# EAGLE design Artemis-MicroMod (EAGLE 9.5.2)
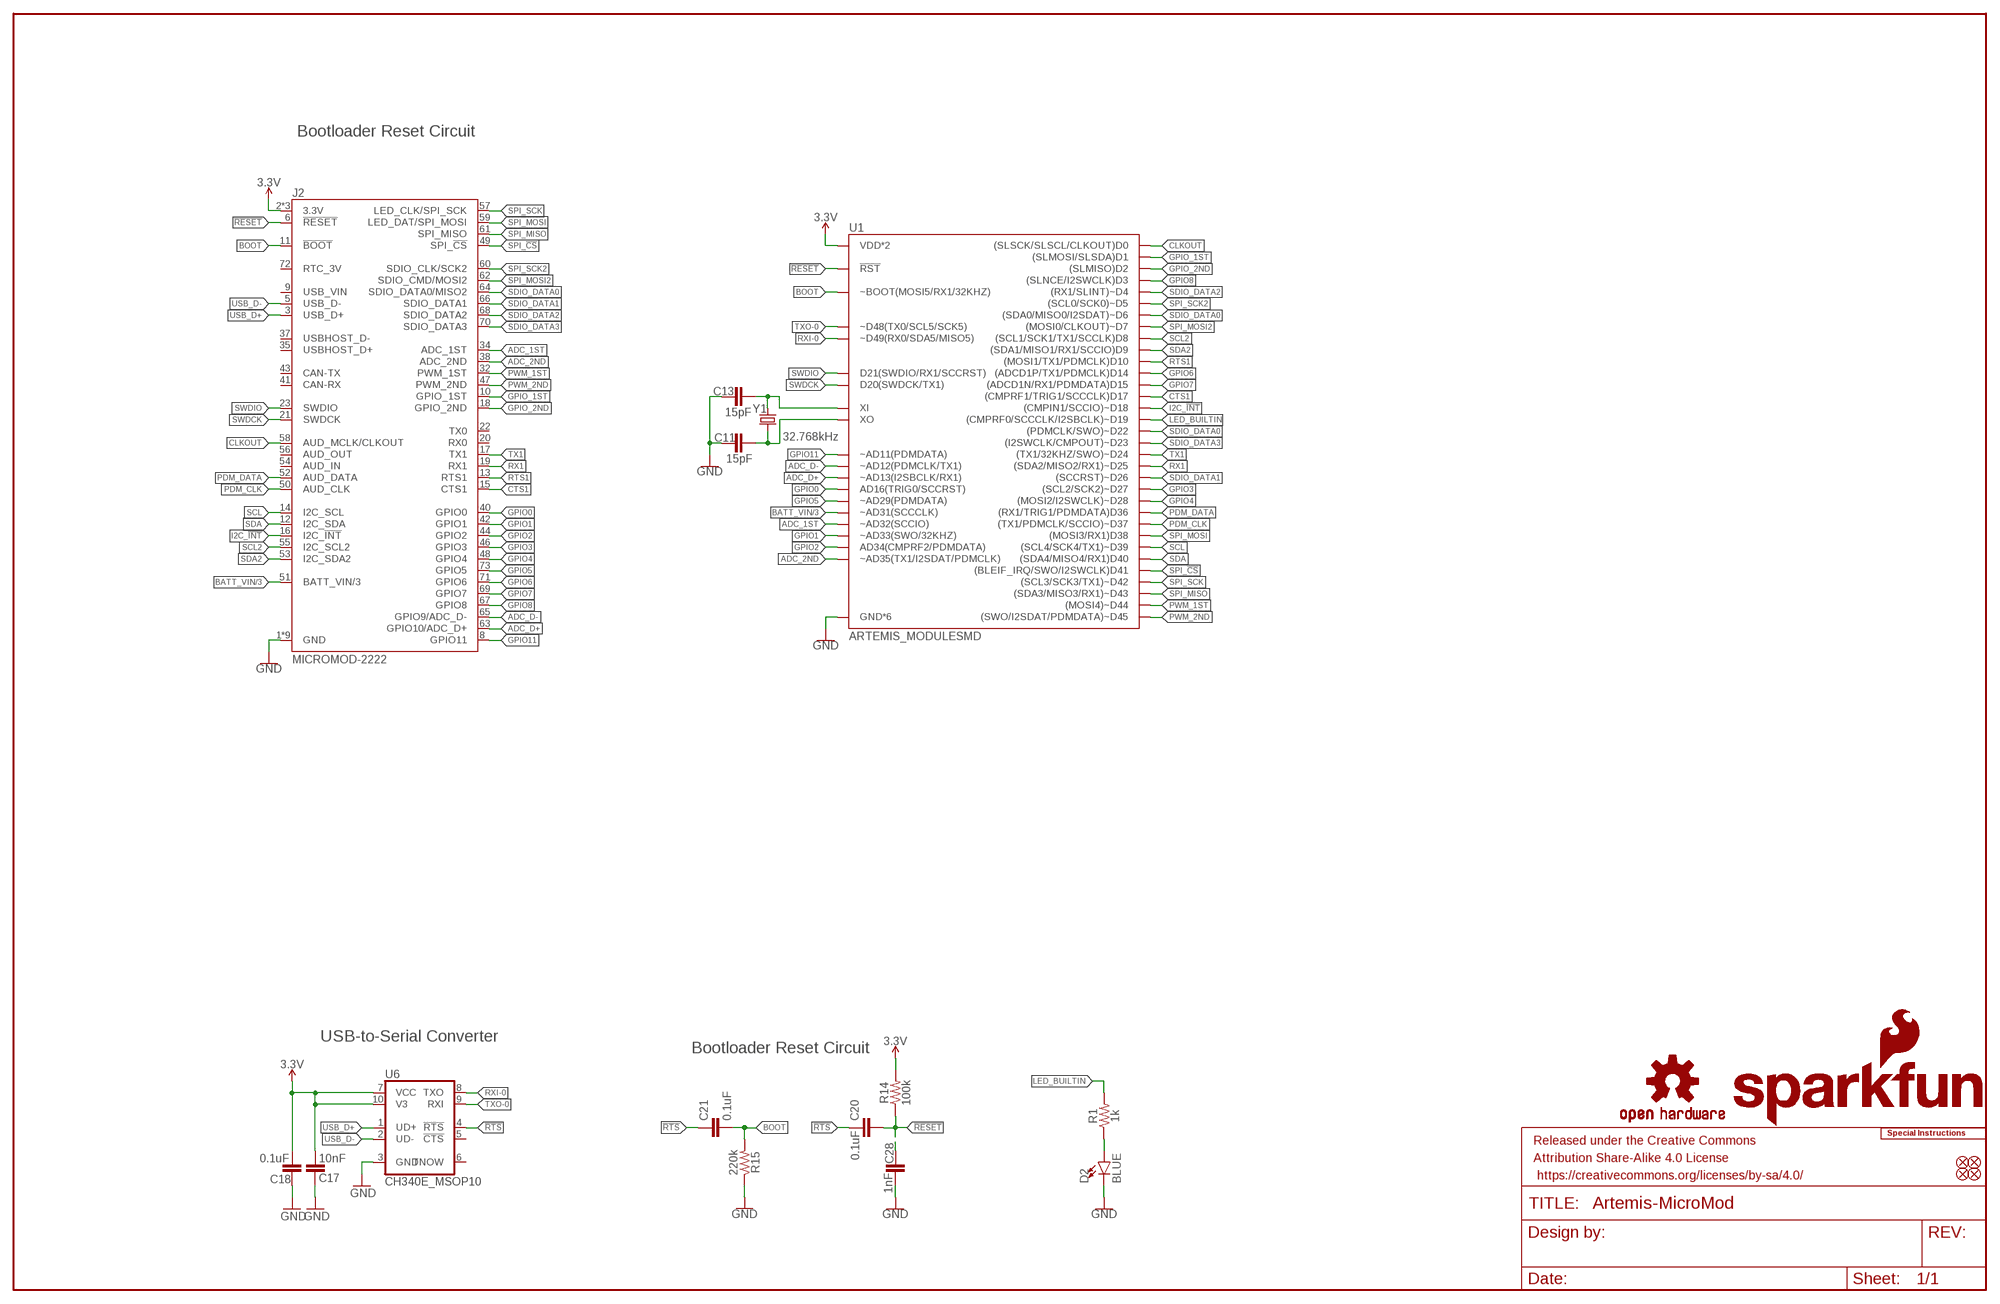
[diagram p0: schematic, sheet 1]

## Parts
C11  15pF  15PF-0603-50V-5%  [0603]
C13  15pF  15PF-0603-50V-5%  [0603]
C17  10nF  10NF-0603-50V-10%  [0603]
C18  0.1uF  0.1UF-0603-25V-(+80/-20%)  [0603]
C20  0.1uF  0.1UF-0603-25V-5%  [0603]
C21  0.1uF  0.1UF-0603-25V-5%  [0603]
C28  1nF  1.0NF/1000PF-0603-50V-10%  [0603]
D2  BLUE  LED-BLUE0603  [LED-0603]
FD1  FIDUCIALUFIDUCIAL  [FIDUCIAL-MICRO]
FD2  FIDUCIALUFIDUCIAL  [FIDUCIAL-MICRO]
FD3  FIDUCIALUFIDUCIAL  [FIDUCIAL-MICRO]
FD4  FIDUCIALUFIDUCIAL  [FIDUCIAL-MICRO]
FRAME1  FRAME-LEDGER  [CREATIVE_COMMONS]
J2  MICROMOD-2222  [M.2-CARD-E-22]
LOGO1  SFE_LOGO_NAME_FLAME.1_INCH  [SFE_LOGO_NAME_FLAME_.1]
LOGO2  SFE_LOGO_FLAME.1_INCH  [SFE_LOGO_FLAME_.1]
LOGO3  OSHW-LOGOMINI  [OSHW-LOGO-MINI]
LOGO4  SPECIAL_INSTRUCTIONS-ORDERING  [ORDERING_INSTRUCTIONS]
R1  1k  1KOHM-0603-1/10W-1%  [0603]
R14  100k  100KOHM-0603-1/10W-1%  [0603]
R15  220k  220KOHM-0603-1/10W-1%  [0603]
U1  ARTEMIS_MODULESMD  [ARTEMIS_FP]
U6  CH340E_MSOP10  [MSOP10]
Y1  32.768kHz  CRYSTAL-32.768KHZSMD-3.2X1.5  [CRYSTAL-SMD-3.2X1.5MM]

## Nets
3.3V: C17.1 C18.1 J2.2(3.3V) J2.4(3.3V) J2.74(3.3V) R14.2 U1.VDD@36(VDD*2) U1.VDD@37(VDD*2) U6.7(VCC) U6.10(V3)
!RESET!: C20.2 C28.1 J2.6(!RESET!) R14.1 U1.~RST(!RST)
!RTS: C20.1 C21.1 U6.4(!RTS)
ADC_1ST: J2.34(ADC_1ST) U1.~AD32(~AD32(SCCIO))
ADC_2ND: J2.38(ADC_2ND) U1.~AD35(~AD35(TX1/I2SDAT/PDMCLK))
ADC_D+: J2.63(GPIO10/ADC_D+) U1.~AD13(~AD13(I2SBCLK/RX1))
ADC_D-: J2.65(GPIO9/ADC_D-) U1.~AD12(~AD12(PDMCLK/TX1))
BATT_VIN/3: J2.51(BATT_VIN/3) U1.~AD31(~AD31(SCCCLK))
BOOT: C21.2 J2.11(!BOOT!) R15.2 U1.BOOT(~BOOT(MOSI5/RX1/32KHZ))
CLKOUT: J2.58(AUD_MCLK/CLKOUT) U1.D0((SLSCK/SLSCL/CLKOUT)D0)
CTS1: J2.15(CTS1) U1.D17((CMPRF1/TRIG1/SCCCLK)D17)
GND: C11.1 C13.1 C17.2 C18.2 C28.2 D2.C J2.1(GND) J2.7(GND) J2.33(GND) J2.36(GND) J2.39(GND) J2.45(GND) J2.75(GND) J2.GND J2.GND-SM-B(GND) R15.1 U1.GND@1(GND*6) U1.GND@22(GND*6) U1.GND@38(GND*6) U1.GND@39(GND*6) U1.GND@47(GND*6) U1.GND@59(GND*6) U6.3(GND)
GPIO0: J2.40(GPIO0) U1.AD16(AD16(TRIG0/SCCRST))
GPIO1: J2.42(GPIO1) U1.~AD33/SWO(~AD33(SWO/32KHZ))
GPIO2: J2.44(GPIO2) U1.AD34(AD34(CMPRF2/PDMDATA))
GPIO3: J2.46(GPIO3) U1.~D27((SCL2/SCK2)~D27)
GPIO4: J2.48(GPIO4) U1.~D28((MOSI2/I2SWCLK)~D28)
GPIO5: J2.73(GPIO5) U1.~AD29(~AD29(PDMDATA))
GPIO6: J2.71(GPIO6) U1.D14((ADCD1P/TX1/PDMCLK)D14)
GPIO7: J2.69(GPIO7) U1.D15((ADCD1N/RX1/PDMDATA)D15)
GPIO8: J2.67(GPIO8) U1.D3((SLNCE/I2SWCLK)D3)
GPIO11: J2.8(GPIO11) U1.~AD11(~AD11(PDMDATA))
GPIO_1ST: J2.10(GPIO_1ST) U1.D1((SLMOSI/SLSDA)D1)
GPIO_2ND: J2.18(GPIO_2ND) U1.D2((SLMISO)D2)
I2C_!INT!: J2.16(I2C_!INT!) U1.~D18((CMPIN1/SCCIO)~D18)
LED_BUILTIN: R1.2 U1.~D19((CMPRF0/SCCCLK/I2SBCLK)~D19)
N$2: D2.A R1.1
N$7: C11.2 U1.XO Y1.P$2
N$8: C13.2 U1.XI Y1.P$1
PDM_CLK: J2.50(AUD_CLK) U1.~D37((TX1/PDMCLK/SCCIO)~D37)
PDM_DATA: J2.52(AUD_DATA) U1.D36((RX1/TRIG1/PDMDATA)D36)
PWM_1ST: J2.32(PWM_1ST) U1.~D44((MOSI4)~D44)
PWM_2ND: J2.47(PWM_2ND) U1.~D45((SWO/I2SDAT/PDMDATA)~D45)
RTS1: J2.13(RTS1) U1.D10((MOSI1/TX1/PDMCLK)D10)
RX1: J2.19(RX1) U1.~D25((SDA2/MISO2/RX1)~D25)
RXI-0: U1.RXI-0(~D49(RX0/SDA5/MISO5)) U6.8(TXO)
SCL: J2.14(I2C_SCL) U1.~D39((SCL4/SCK4/TX1)~D39)
SCL2: J2.55(I2C_SCL2) U1.D8((SCL1/SCK1/TX1/SCCLK)D8)
SDA: J2.12(I2C_SDA) U1.D40((SDA4/MISO4/RX1)D40)
SDA2: J2.53(I2C_SDA2) U1.D9((SDA1/MISO1/RX1/SCCIO)D9)
SDIO_DATA0: J2.64(SDIO_DATA0/MISO2) U1.~D6((SDA0/MISO0/I2SDAT)~D6) U1.~D22((PDMCLK/SWO)~D22)
SDIO_DATA1: J2.66(SDIO_DATA1) U1.~D26((SCCRST)~D26)
SDIO_DATA2: J2.68(SDIO_DATA2) U1.~D4((RX1/SLINT)~D4)
SDIO_DATA3: J2.70(SDIO_DATA3) U1.~D23((I2SWCLK/CMPOUT)~D23)
SPI_!CS!: J2.49(SPI_!CS!) U1.D41((BLEIF_IRQ/SWO/I2SWCLK)D41)
SPI_MISO: J2.61(SPI_MISO) U1.~D43((SDA3/MISO3/RX1)~D43)
SPI_MOSI: J2.59(LED_DAT/SPI_MOSI) U1.D38((MOSI3/RX1)D38)
SPI_MOSI2: J2.62(SDIO_CMD/MOSI2) U1.D7((MOSI0/CLKOUT)~D7)
SPI_SCK: J2.57(LED_CLK/SPI_SCK) U1.~D42((SCL3/SCK3/TX1)~D42)
SPI_SCK2: J2.60(SDIO_CLK/SCK2) U1.~D5((SCL0/SCK0)~D5)
SWDCK: J2.21(SWDCK) U1.SWDCK(D20(SWDCK/TX1))
SWDIO: J2.23(SWDIO) U1.SWDIO(D21(SWDIO/RX1/SCCRST))
TX1: J2.17(TX1) U1.~D24((TX1/32KHZ/SWO)~D24)
TXO-0: U1.TXO-0(~D48(TX0/SCL5/SCK5)) U6.9(RXI)
USB_D+: J2.3(USB_D+) U6.1(UD+)
USB_D-: J2.5(USB_D-) U6.2(UD-)
Unconnected: J2.9(USB_VIN) J2.20(RX0) J2.22(TX0) J2.35(USBHOST_D+) J2.37(USBHOST_D-) J2.41(CAN-RX) J2.43(CAN-TX) J2.54(AUD_IN) J2.56(AUD_OUT) J2.72(RTC_3V) U6.5(!CTS) U6.6(TNOW)

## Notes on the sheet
- Bootloader Reset Circuit
- USB-to-Serial Converter
- Bootloader Reset Circuit

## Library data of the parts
C11 C13 = SparkFun-Capacitors:15PF: 15pF ceramic capacitors; PROD_ID: CAP-07881
C17 = SparkFun-Capacitors:10NF: 0.01uF/10nF/10,000pF ceramic capacitors; PROD_ID: CAP-00867
C18 = SparkFun-Capacitors:0.1UF: 0.1µF ceramic capacitors; PROD_ID: CAP-00810
C20 C21 = SparkFun-Capacitors:0.1UF: 0.1µF ceramic capacitors; PROD_ID: CAP-08604
C28 = SparkFun-Capacitors:1.0NF/1000PF: 1nF/1,000pF ceramic capacitors; PROD_ID: CAP-07886
D2 = SparkFun-LED:LED-BLUE: Blue SMD LED; PROD_ID: DIO-08575
FD1-FD4 = SparkFun-Aesthetics:FIDUCIAL: Fiducial Alignment Points
FRAME1 = SparkFun-Aesthetics:FRAME-LEDGER: Schematic Frame - Ledger
J2 = Teensy:MICROMOD
LOGO1 = SparkFun-Aesthetics:SFE_LOGO_NAME_FLAME: SparkFun Font Logo w/ Flame
LOGO2 = SparkFun-Aesthetics:SFE_LOGO_FLAME: SparkFun Flame Logo
LOGO3 = SparkFun-Aesthetics:OSHW-LOGO: Open-Source Hardware (OSHW) Logo
LOGO4 = SparkFun-Aesthetics:SPECIAL_INSTRUCTIONS: Special Ordering/Production Instructions Alert
R1 = SparkFun-Resistors:1KOHM: 1kΩ resistor; PROD_ID: RES-07856
R14 = SparkFun-Resistors:100KOHM: 100kΩ resistor; PROD_ID: RES-07828
R15 = SparkFun-Resistors:220KOHM: 220kΩ resistor; PROD_ID: RES-08969
U1 = SparkFun-IC-Microcontroller:ARTEMIS_MODULE: Description: The Artemis Module from SparkFun is a Cortex-M4F with BLE 5.0 running up to 96MHz and with as low power as 6uA per MHz (less than 5mW). This is the world's first module to bridge the market between hobbyists and consumer products. We've packaged all the power of a modern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; PROD_ID: SUB-14402
U6 = SparkFun-IC-Comms:CH340E; PROD_ID: IC-14135
Y1 = SparkFun-Clocks:CRYSTAL-32.768KHZ: 32.768kHz Crystal; PROD_ID: XTAL-13062

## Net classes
0 default: width 0 mm, drill 0 mm

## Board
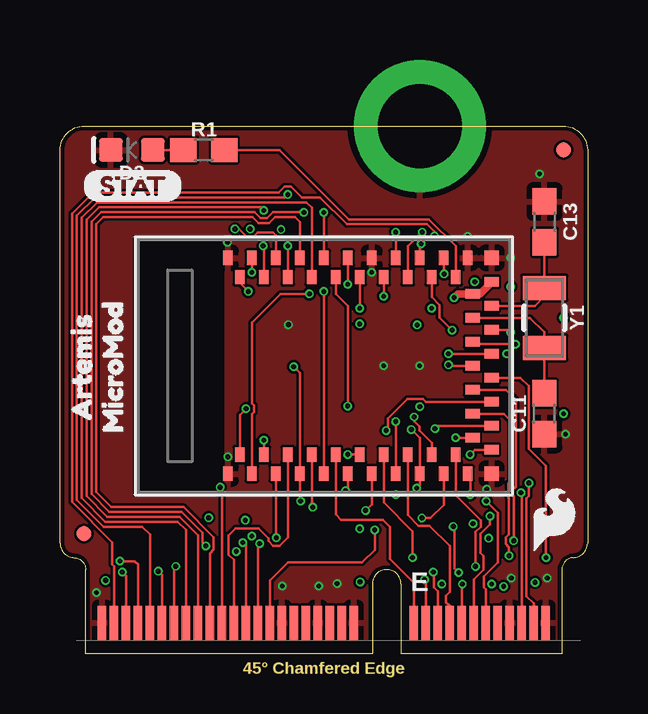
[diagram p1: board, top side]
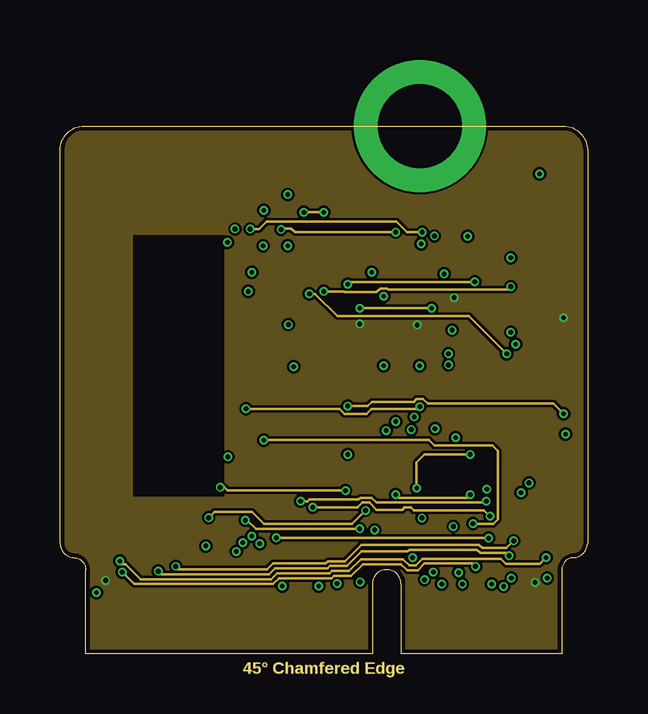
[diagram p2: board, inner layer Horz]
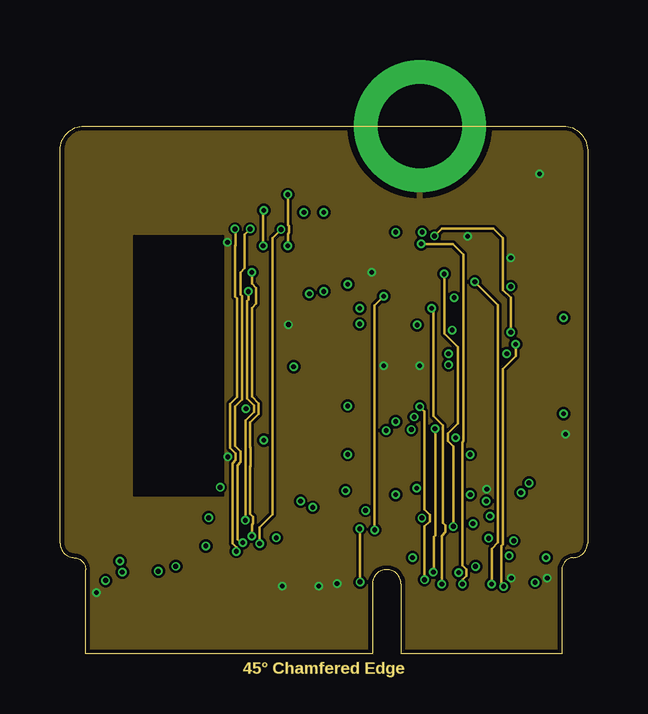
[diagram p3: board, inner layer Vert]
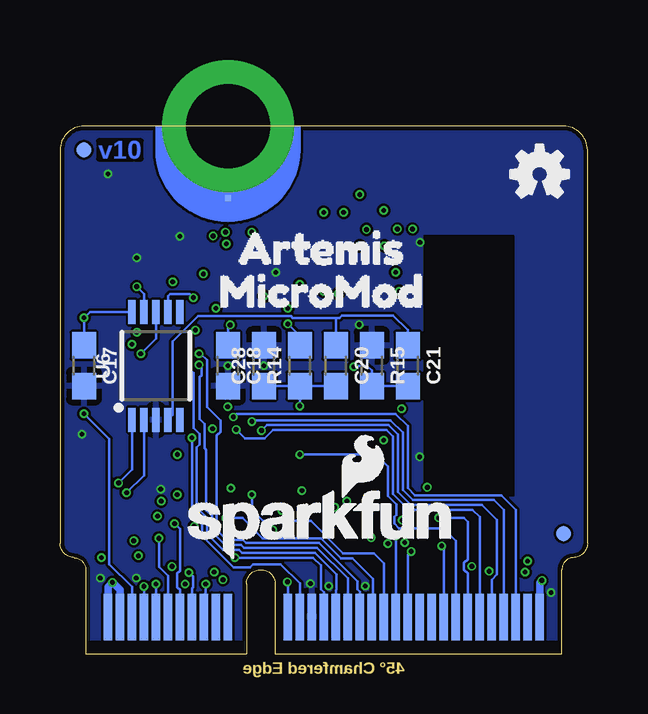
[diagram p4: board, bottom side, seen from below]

Size 22 x 22 mm. Coordinates in mm from the lower left corner, seen from the top.
Outline: 0,4.6 0,21 arc-87 1,22 21,22 arc-87 22,21 22,4.6
Outline: 0,4.6 arc87 0.6,4
Outline: 21.4,4 arc87 22,4.6
Outline: 21.4,4 arc85 20.93,3.5 20.93,0 14.22,0 14.22,2.9 arc180 13.03,2.9 13.03,0 1.07,0 1.07,3.5 arc84 0.6,4
Outline: 21.4,4 arc87 22,4.6
Outline: 0,4.6 arc87 0.6,4
Copper layers (1+2*15+16): Top 0.035mm / dielectric 1.5mm / Horz 0.035mm / dielectric 0.15mm / Vert 0.035mm / dielectric 0.2mm / Bottom 0.035mm
Design rules "SparkFun-4-layer-MicroMod": minimum track width 4mil, minimum drill 0.2mm, track to track 4mil, track to pad 4mil, pad to pad 4mil, via to via 4mil, smd to smd 4mil, copper to edge 6mil, drill to drill 6mil, minimum pad ring 3mil, minimum via ring 3mil, stop-mask expansion 4mil, vias tented up to drill 25mil, thermal gap 10mil
tKeepout: area 3.1,6.6 to 6.6,17.3

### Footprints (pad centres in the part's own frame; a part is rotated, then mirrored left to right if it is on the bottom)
0603 = smd 1.1 x 1: 1 -0.85,0; 2 0.85,0
LED-0603 = smd 1 x 1: A -0.877,0; C 0.877,0
FIDUCIAL-MICRO = smd 0.635 x 0.635: 1 0,0
M.2-CARD-E-22 = smd 0.35 x 1.45: 1 9.25,1.275; 3 8.75,1.275; 5 8.25,1.275; 7 7.75,1.275; 9 7.25,1.275; 11 6.75,1.275; 13 6.25,1.275; 15 5.75,1.275; 17 5.25,1.275; 19 4.75,1.275; 21 4.25,1.275; 23 3.75,1.275; 33 1.25,1.275; 35 0.75,1.275; 37 0.25,1.275; 39 -0.25,1.275; 41 -0.75,1.275; 43 -1.25,1.275; 45 -1.75,1.275; 47 -2.25,1.275; 49 -2.75,1.275; 51 -3.25,1.275; 53 -3.75,1.275; 55 -4.25,1.275; 57 -4.75,1.275; 59 -5.25,1.275; 61 -5.75,1.275; 63 -6.25,1.275; 65 -6.75,1.275; 67 -7.25,1.275; 69 -7.75,1.275; 71 -8.25,1.275; 73 -8.75,1.275; 75 -9.25,1.275 | smd 0.35 x 1.95 bottom: 2 9,1.525; 4 8.5,1.525; 6 8,1.525; 8 7.5,1.525; 10 7,1.525; 12 6.5,1.525; 14 6,1.525; 16 5.5,1.525; 18 5,1.525; 20 4.5,1.525; 22 4,1.525; 32 1.5,1.525; 34 1,1.525; 36 0.5,1.525; 38 0,1.525; 40 -0.5,1.525; 42 -1,1.525; 44 -1.5,1.525; 46 -2,1.525; 48 -2.5,1.525; 50 -3,1.525; 52 -3.5,1.525; 54 -4,1.525; 56 -4.5,1.525; 58 -5,1.525; 60 -5.5,1.525; 62 -6,1.525; 64 -6.5,1.525; 66 -7,1.525; 68 -7.5,1.525; 70 -8,1.525; 72 -8.5,1.525; 74 -9,1.525 | drill 3.5 pad 5.5: GND 4,22 | smd 0.25 x 0.25 bottom: GND-SM-B 4,19
ARTEMIS_FP = smd 0.4 x 0.6: AD16 -4,-3.7; BOOT 1.5,4.5; D0 0.5,-4.5; D1 -0.5,-4.5; D2 -1,-3.7; D3 2,-3.7; D7 -1.5,4.5; D8 -0.5,4.5; D9 2,3.7; D10 1,3.7; D14 -5,3.7; D17 -3.5,-4.5; D36 2.5,-4.5; D38 3,-3.7; D40 2.5,4.5; D41 -2.5,-4.5; GND@1 4.5,4.5; GND@39 -5.5,-4.5; GND@47 -1.5,-4.5; GND@59 4.5,-4.5; RXI-0 3.5,4.5; SWDCK 4,3.7; SWDIO 0,3.7; TXO-0 0.5,4.5; ~AD31 -3,-3.7; ~AD35 -2,3.7; ~D4 -2.5,4.5; ~D5 -1,3.7; ~D18 -4.5,-4.5; ~D19 -5,-3.7; ~D22 -3.5,4.5; ~D23 -4,3.7; ~D24 -3,3.7; ~D27 -4.5,4.5; ~D28 -5.5,4.5; ~D37 3.5,-4.5; ~D39 3,3.7; ~D42 1.5,-4.5; ~D43 1,-3.7; ~D44 4,-3.7; ~D45 -2,-3.7; ~RST 0,-3.7 | smd 0.6 x 0.4: AD34 -6.5,-0.5; D15 -6.5,0.5; VDD@36 -5.7,-3; VDD@37 -6.5,-3.5; XI -6.5,-2.5; XO -5.7,-2; ~AD11 -5.7,-1; ~AD12 -5.7,2; ~AD13 -5.7,1; ~AD29 -6.5,-1.5; ~AD32 -5.7,3; ~AD33/SWO -5.7,0; ~D6 -6.5,3.5; ~D25 -6.5,2.5; ~D26 -6.5,1.5 | smd 0.6 x 0.6: GND@22 -6.5,4.5; GND@38 -6.5,-4.5
MSOP10 = smd 1 x 0.3: 1 -2.25,1; 2 -2.25,0.5; 3 -2.25,0; 4 -2.25,-0.5; 5 -2.25,-1; 6 2.25,-1; 7 2.25,-0.5; 8 2.25,0; 9 2.25,0.5; 10 2.25,1
CRYSTAL-SMD-3.2X1.5MM = smd 1 x 1.8: P$1 -1.25,0; P$2 1.25,0

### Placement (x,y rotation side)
C11  20.2,10 90 top
C13  20.2,18 270 top
C17  21,12 270 bottom
C18  15,12 270 bottom
C20  10.5,12 270 bottom
C21  7.5,12 270 bottom
C28  13.5,12 90 bottom
D2  3,21 180 top
FD1  1,5 0 top
FD2  21,21 0 top
FD3  21,21 0 bottom
FD4  1,5 0 bottom
FRAME1  not placed on the board
J2  11,0 0 top
LOGO1  11.1,5.4 0 bottom
LOGO2  20.6,5.6 0 top
LOGO3  2,20 0 bottom
LOGO4  not placed on the board
R1  6,21 0 top
R14  12,12 90 bottom
R15  9,12 270 bottom
U1  11.5,12 180 top
U6  18,12 90 bottom
U$1  [STAT_32]  0.9,19.5 0 top
U$2  [ARTEMIS0]  0.9,9 90 top
U$3  [MICROMOD1]  2.2,8.5 90 top
U$6  [ARTEMIS2]  15.7,16.9 0 bottom
U$7  [MICROMOD1]  16.5,15.1 0 bottom
Y1  20.2,14 270 top

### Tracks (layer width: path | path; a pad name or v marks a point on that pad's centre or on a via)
3.3V  (via drill 0.2)
  Top 0.305: U1.VDD@37 17.5,15 U1.VDD@36 16.59,15 v16.43,14.84
  Bottom 0.102: C17.1 v21,14 20.75,14.25 U6.10 | U6.7 17.5,14.9 17.4,15 16.59,15 v16.43,14.84 | R14.2 12,13.24 v12.5,13.74 | C18.1 15,13.6 v14.9,13.7
  Bottom 0.305: J2.2 20,2.78 v19.81,2.97 19.5,2.65 J2.4 | J2.74 2,2.95 v1.91,3.05
  pour Horz (isolate 0.102): 0,22 22,22 22,0 0,0
!RESET!  (via drill 0.2)
  Top 0.102: U1.~RST 11.5,15 12,14.5 v12,10.32
  Horz 0.102: v21,10 20.58,10.42 15.34,10.42 15.14,10.62 14.87,10.62 14.75,10.5 13,10.5 12.82,10.32 v12,10.32
  Bottom 0.102: R14.1 C28.1 | R14.1 C20.2 | J2.6 19,2.79 19.94,3.73 19.94,8.94 v21,10 | R14.1 v12,10.32
!RTS
  Bottom 0.102: C21.1 7.5,13.48 8.11,14.1 10.24,14.1 10.34,14 10.5,14 | U6.4 17.3,9.95 17.3,13 16.23,14.07 12.36,14.07 12.29,14 10.5,14 | C20.1 10.5,14
ADC_1ST  (via drill 0.2)
  Top 0.102: v16.5,9 U1.~AD32
  Bottom 0.102: J2.34 12,2.94 12.79,3.73 13.94,3.73 14.07,3.6 14.77,3.6 16.08,4.91 16.08,5.58 16.5,6 v16.5,9
ADC_2ND  (via drill 0.2)
  Top 0.102: U1.~AD35 13.5,6.3 14.7,5.1 v14.7,4
  Bottom 0.102: v14.7,4 14.49,4 14.48,4 11.45,4 11.12,3.67 11.12,2.68 11,2.55 J2.38
ADC_D+  (via drill 0.2)
  Top 0.102: J2.63 4.75,3.56 v4.83,3.63 | U1.~AD13 18.6,11 19,10.6 19,6.95 18.89,6.85 18.89,6.58 18.92,6.55 v18.92,4.7
  Horz 0.102: v4.83,3.63 4.95,3.51 8.64,3.51 8.88,3.75 11.07,3.75 11.17,3.85 11.89,3.85 12.57,4.53 17.48,4.53 17.61,4.4 18.62,4.4 v18.92,4.7
ADC_D-  (via drill 0.2)
  Top 0.102: v4.1,3.43 4.25,3.28 J2.65 | v18.73,4.08 18.73,4.43 18.59,4.56 18.59,4.84 18.72,4.96 18.72,6.46 18.69,6.49 18.69,7.09 18.8,7.2 18.8,9.7 18.5,10 U1.~AD12
  Horz 0.102: v4.1,3.43 4.22,3.31 8.72,3.31 8.97,3.55 11.15,3.55 11.25,3.65 11.97,3.65 12.58,4.25 14.49,4.25 14.56,4.33 17.39,4.33 17.52,4.2 18.7,4.2 18.73,4.17 v18.73,4.08
BATT_VIN/3  (via drill 0.2)
  Top 0.102: J2.51 7.75,4.51 v7.63,4.63 | v15.1,17.57 14.94,17.41 14.93,17.41 14.5,16.98 U1.~AD31
  Horz 0.102: v15.1,17.57 14.46,17.57 14.03,18.01 8.62,18.01 8.31,17.7 v7.93,17.7
  Vert 0.102: v7.93,17.7 7.7,17.47 7.7,16.07 7.53,15.89 7.53,14.96 7.6,14.9 7.6,10.6 7.3,10.3 7.3,8.65 7.53,8.42 7.53,7.98 7.4,7.85 7.4,4.75 7.53,4.63 v7.63,4.63
BOOT  (via drill 0.2)
  Top 0.102: v9.74,11.96 10,11.7 U1.BOOT 10,6.38 v10.03,6.35 | v17.78,6.35 v17.78,6.34 18.26,5.86 18.26,3.81 17.67,3.22 17.67,2.76 17.75,2.69 J2.11
  Horz 0.102: v10.03,6.35 10.33,6.35 10.4,6.42 12.45,6.42 12.52,6.5 12.99,6.5 13.19,6.3 17.73,6.3 v17.78,6.35
  Bottom 0.102: C21.2 R15.2 9,11.8 9.2,12 9.7,12 v9.74,11.96
CLKOUT  (via drill 0.2)
  Top 0.102: v6.08,4.48 5.95,4.62 5.95,5.02 5.07,5.91 2.06,5.91 1.31,6.65 1.31,18 1.72,18.4 8.11,18.4 8.36,18.15 8.64,18.15 8.89,18.4 v10.17,18.4 | v11,18.4 U1.D0
  Horz 0.102: v10.17,18.4 v11,18.4
  Bottom 0.102: J2.58 6,4.4 v6.08,4.48
CTS1  (via drill 0.2)
  Top 0.102: U1.D17 15,17.08 v15.06,17.08 | J2.15 16.75,2.9 v16.78,2.9
  Vert 0.102: v15.06,17.08 16.38,17.08 16.83,16.64 16.83,8.86 16.77,8.81 16.77,8.16 16.78,8.15 16.78,3.68 16.95,3.51 16.95,3.24 16.78,3.07 v16.78,2.9
GND  (via drill 0.2)
  other vias: 20.32,3.15 21.08,9.14 17.8,6.86 15,12 13.5,12 9.53,13.72 6.99,17.14 1.52,2.54 7,8.2 9.27,2.81 10.79,2.81 11.56,2.91 18.82,3.15 20,20 13,15.9 18.8,16.5 17,17.4
  pour Top (isolate 0.102): 0,22 22,22 22,0.6 0,0.6
  pour Bottom (isolate 0.102): 0,22 22,22 22,0.6 0,0.6
  pour Vert (isolate 0.102): 0,22 22,22 22,0 0,0
  cutout Bottom (isolate 0.102): 3.1,17.4 6.8,17.4 6.8,6.6 3.1,6.6
  cutout Horz (isolate 0.102): 3.1,17.4 6.8,17.4 6.8,6.6 3.1,6.6
  cutout Vert (isolate 0.102): 3.1,17.4 6.8,17.4 6.8,6.6 3.1,6.6
  cutout Top (isolate 0.102): 3.1,17.4 6.8,17.4 6.8,6.6 3.1,6.6
GPIO0  (via drill 0.2)
  Top 0.102: v16.35,13.49 15.83,14.01 15.83,14.54 15.5,14.87 U1.AD16
  Bottom 0.102: v16.35,13.49 16.53,13.31 16.53,11.8 16.43,11.7 16.43,9.41 16.17,9.16 16.17,8.73 16.3,8.6 16.3,6.08 15.87,5.66 15.87,5 15.21,4.33 14.53,4.33 14.4,4.2 11.36,4.2 10.47,3.3 10.47,2.68 10.5,2.64 J2.40
GPIO1  (via drill 0.2)
  Top 0.102: U1.~AD33/SWO 16.23,12 v16.2,12.04
  Bottom 0.102: v16.2,12.04 16.1,12.04 16.1,11.6 16.17,11.53 16.17,9.77 15.97,9.57 15.97,8.57 15.9,8.5 15.9,5.97 15.66,5.74 15.66,5.07 15.12,4.53 14.44,4.53 14.32,4.4 11.28,4.4 10,3.12 J2.42
GPIO2  (via drill 0.2)
  Top 0.102: U1.AD34 v16.2,12.5
  Bottom 0.102: v16.2,12.5 16.14,12.5 15.87,12.24 15.87,10.28 15.31,9.71 15.31,9.24 15.46,9.09 15.46,5.16 15.15,4.85 15.04,4.74 14.36,4.74 14.23,4.61 11.19,4.61 9.6,3.01 9.6,2.68 9.5,2.58 J2.44
GPIO3  (via drill 0.2)
  Top 0.102: U1.~D27 16,6.2 15.45,5.65 v15.09,5.65
  Bottom 0.102: J2.46 9,2.22 8.94,2.28 8.94,3.12 9.8,3.98 10.28,3.98 11.11,4.81 13.55,4.81 14.39,5.65 v15.09,5.65
GPIO4  (via drill 0.2)
  Top 0.102: U1.~D28 17.11,7.39 v17.11,6.62
  Horz 0.102: v17.11,6.62 16.98,6.5 14.12,6.5 v14,6.62
  Bottom 0.102: J2.48 8.5,3.76 8.92,4.18 10.19,4.18 11.54,5.53 13.53,5.53 14,6 v14,6.62
GPIO5  (via drill 0.2)
  Top 0.102: J2.73 2.25,3.64 2.17,3.72 2.17,4.64 0.5,6.32 0.5,18.34 1.38,19.22 9.11,19.22 9.36,19.47 9.64,19.47 10.09,19.01 10.85,19.01 11.96,17.9 15.3,17.9 15.61,17.59 v15.61,17.41 | U1.~AD29 18.7,13.5 v18.8,13.4
  Vert 0.102: v18.8,13.4 18.8,14.84 18.47,15.16 18.47,17.33 18.07,17.73 15.93,17.73 v15.61,17.41
GPIO6  (via drill 0.2)
  Top 0.102: J2.71 2.75,3.25 v2.6,3.4 | v17.33,3.63 17.33,5.06 17.55,5.28 17.55,5.56 16.5,6.6 U1.D14
  Horz 0.102: v2.6,3.4 3.1,2.9 8.89,2.9 9.13,3.14 11.32,3.14 11.42,3.24 12.14,3.24 12.63,3.73 14.22,3.73 14.48,3.47 14.92,3.47 15.21,3.75 17.2,3.75 v17.33,3.63
GPIO7  (via drill 0.2)
  Top 0.102: J2.69 3.25,3.71 3.11,3.85 v2.5,3.85 | U1.D15 19.2,11.5 19.55,11.15 19.55,8.54 20.27,7.82 v20.27,4
  Horz 0.102: v2.5,3.85 2.62,3.73 2.74,3.73 3.36,3.1 8.81,3.1 9.05,3.35 11.24,3.35 11.34,3.44 12.06,3.44 12.54,3.93 14.3,3.93 14.56,3.67 14.84,3.67 15.12,3.96 18.38,3.96 18.59,3.75 20.01,3.75 v20.27,4
GPIO8  (via drill 0.2)
  Top 0.102: J2.67 3.75,4.97 3.44,5.28 1.82,5.28 0.7,6.4 0.7,18.25 1.46,19.01 9.38,19.01 v9.5,19.14 | v9.5,17 U1.D3
  Vert 0.102: v9.5,19.14 9.5,17.86 9.55,17.82 9.55,17.55 9.5,17.5 v9.5,17
GPIO11  (via drill 0.2)
  Top 0.102: v19,12.9 17.3,12.9 U1.~AD11
  Vert 0.102: v18.5,2.8 18.4,2.9 18.4,4.48 18.46,4.54 18.46,11.86 19,12.4 v19,12.9
  Bottom 0.102: J2.8 v18.5,2.8
GPIO_1ST  (via drill 0.2)
  Top 0.102: v12,15.4 U1.D1
  Horz 0.102: v17.3,15.5 12.1,15.5 v12,15.4
  Vert 0.102: v18,2.9 18,4.37 18.26,4.63 18.26,14.54 v17.3,15.5
  Bottom 0.102: J2.10 v18,2.9
GPIO_2ND  (via drill 0.2)
  Top 0.102: v12.5,14.4 U1.D2
  Horz 0.102: v15.5,14.4 v12.5,14.4
  Vert 0.102: v15.5,14.4 15.57,14.33 15.57,9.91 15.97,9.52 15.97,5.45 16.08,5.34 16.08,5.07 15.92,4.92 v15.92,2.89
  Bottom 0.102: v15.92,2.89 15.92,2.52 16,2.44 J2.18
I2C_!INT!  (via drill 0.2)
  Top 0.102: v16.62,3.38 16.45,3.55 16.45,5.19 16.41,5.24 v16.41,5.3 | v16.02,15.83 16,15.85 U1.~D18
  Vert 0.102: v16.41,5.3 16.41,8.63 16.17,8.86 16.17,9.17 16.6,9.6 16.6,12.78 16.02,13.35 v16.02,15.82 v16.02,15.83
  Bottom 0.102: J2.16 16.5,2.72 16.45,2.76 16.45,3.21 v16.62,3.38
LED_BUILTIN
  Top 0.102: R1.2 9.15,21 12.05,18.1 15.38,18.1 16.5,16.99 U1.~D19
N$2
  Top 0.102: R1.1 D2.A
N$7
  Top 0.102: U1.XO 19.6,14 20.2,13.4 Y1.P$2 C11.2
N$8
  Top 0.102: U1.XI 19.8,14.5 20.2,14.9 Y1.P$1 C13.2
PDM_CLK  (via drill 0.2)
  Top 0.102: v8,15.9 U1.~D37
  Vert 0.102: v8,15.9 8,15.42 8.19,15.24 8.19,14.59 8,14.4 8,10.71 8.29,10.43 8.29,9.99 7.93,9.63 7.93,8.59 7.94,8.59 7.94,7.81 7.93,7.81 7.93,5.82 8.06,5.69 8.06,5.42 8,5.36 v8,4.9
  Bottom 0.102: J2.50 v8,4.9
PDM_DATA  (via drill 0.2)
  Top 0.102: U1.D36 9,17.43 8.89,17.55 8.24,17.55 8.06,17.37 7.79,17.37 7.46,17.7 v7.3,17.7
  Vert 0.102: v7.36,4.26 7.36,4.43 7.2,4.59 7.2,7.94 7.33,8.06 7.33,8.34 7.1,8.56 7.1,10.4 7.39,10.69 7.39,14.81 7.31,14.89 7.31,17.01 7.31,17.69 v7.3,17.7
  Bottom 0.102: J2.52 7.5,4.12 v7.36,4.26
PWM_1ST  (via drill 0.2)
  Top 0.102: U1.~D44 7.5,15.46 v7.86,15.1
  Horz 0.102: v7.73,5.56 7.81,5.56 8.17,5.2 12.26,5.2 v12.5,5.2
  Vert 0.102: v7.86,15.1 7.86,14.76 7.8,14.7 7.8,10.63 8.09,10.34 8.09,10.07 7.73,9.72 7.73,8.51 7.74,8.5 7.74,7.9 7.73,7.89 v7.73,5.56 | v12.52,2.98 12.52,5.18 v12.5,5.2
  Bottom 0.102: J2.32 12.5,2.97 v12.52,2.98
PWM_2ND  (via drill 0.2)
  Top 0.102: J2.47 8.75,3.05 9.5,3.8 12.6,3.8 13.13,4.33 v13.13,5.16 | v13.5,14.9 U1.~D45
  Vert 0.102: v13.13,5.16 13.11,5.17 13.11,14.51 v13.5,14.9
RTS1  (via drill 0.2)
  Top 0.102: U1.D10 10.5,6.14 v10.54,6.1 | J2.13 17.25,3.09 17.66,3.49 17.66,4.07 17.53,4.19 17.53,4.98 17.93,5.38 v17.93,5.73
  Horz 0.102: v17.93,5.73 17.68,5.98 14.75,5.98 14.64,6.09 14.36,6.09 14.27,6 13.2,6 12.9,6.3 12.61,6.3 12.41,6.1 v10.54,6.1
RX1  (via drill 0.2)
  Top 0.102: v15.64,9.38 15.76,9.5 U1.~D25 | J2.19 15.75,2.6 15.59,2.76 15.59,3.38 v15.57,3.4
  Vert 0.102: v15.57,3.4 15.59,3.4 15.59,4.87 15.65,4.93 v15.65,9.37 v15.64,9.38
RXI-0  (via drill 0.2)
  Top 0.102: U1.RXI-0 8,9.98 8.09,10.07 8.09,10.34 8,10.43 8,13.8 9.2,15 v10.4,15
  Horz 0.102: v10.4,15 10.63,15 11.56,14.07 17.06,14.07 v18.63,12.5
  Bottom 0.102: v18.63,12.5 18,13.13 U6.8
SCL  (via drill 0.2)
  Top 0.102: v8.5,8.9 U1.~D39
  Horz 0.102: v8.5,8.9 15.38,8.9 15.61,8.67 18.03,8.67 18.26,8.44 18.26,5.59 18.07,5.4 17.24,5.4 v17.22,5.42
  Bottom 0.102: v17.22,5.42 17,5.2 17,3.45 17.11,3.34 17.11,2.76 17,2.65 J2.14
SCL2  (via drill 0.2)
  Top 0.102: v11.91,6.79 12,6.88 U1.D8 | v6.68,6.93 6.75,6.86 J2.55
  Horz 0.102: v11.91,6.79 6.99,6.79 6.86,6.93 v6.68,6.93
SDA  (via drill 0.2)
  Top 0.102: U1.D40 9,4.84 v9.02,4.83
  Horz 0.102: v17.87,4.81 17.85,4.83 v9.02,4.83
  Bottom 0.102: v17.87,4.81 17.87,3.61 17.5,3.24 J2.12
SDA2
  Top 0.102: J2.53 7.25,3.9 7.03,4.12 7.03,4.93 7.33,5.23 8.27,5.23 8.69,4.81 8.69,4.69 8.88,4.5 9.15,4.5 9.5,4.84 U1.D9
SDIO_DATA0  (via drill 0.2)
  Top 0.102: v14.65,9.34 15,8.99 U1.~D22 15,7.03 v14.87,6.9 | U1.~D6 17.3,8.5 v17.1,8.3
  Horz 0.102: v17.1,8.3 15.2,8.3 14.87,7.97 v14.87,6.9
  Bottom 0.102: J2.64 4.5,5.69 4.8,5.99 7.45,5.99 8.11,6.65 8.11,9.05 8.38,9.32 13.11,9.32 13.46,8.97 14.29,8.97 v14.65,9.34
SDIO_DATA1  (via drill 0.2)
  Top 0.102: v13.6,9.3 13.67,9.37 13.67,9.81 14.48,10.62 15.14,10.62 15.27,10.5 U1.~D26
  Bottom 0.102: J2.66 4,3.07 3.77,3.3 3.77,5.57 4.4,6.19 7.37,6.19 7.91,6.73 7.91,9.13 8.3,9.53 13.38,9.53 v13.6,9.3
SDIO_DATA2  (via drill 0.2)
  Top 0.102: v14,9.67 U1.~D4
  Bottom 0.102: J2.68 3.5,6 3.9,6.4 7.28,6.4 7.7,6.82 7.7,9.22 8.22,9.73 13.94,9.73 v14,9.67
SDIO_DATA3  (via drill 0.2)
  Top 0.102: U1.~D23 15.5,8.78 14.98,9.3 14.98,9.47 14.77,9.69 v14.77,9.86
  Bottom 0.102: J2.70 3,6 3.6,6.6 7.2,6.6 7.5,6.9 7.5,9.48 8.02,10 11.86,10 11.86,9.99 12.14,9.99 12.14,10 14.63,10 v14.77,9.86
SPI_!CS!  (via drill 0.2)
  Top 0.102: J2.49 8.25,4.51 v8.33,4.59 | U1.D41 v14,17.57
  Horz 0.102: v14,17.57 9.79,17.57 9.64,17.73 9.36,17.73 9.32,17.68 v9.22,17.68
  Vert 0.102: v8.33,4.59 8.33,5.26 8.87,5.8 8.87,17.33 v9.22,17.68
SPI_MISO
  Top 0.102: J2.61 5.25,5.15 4.9,5.5 1.89,5.5 0.91,6.48 0.91,18.17 1.55,18.81 10.29,18.81 10.5,18.6 U1.~D43
SPI_MOSI  (via drill 0.2)
  Top 0.102: J2.59 5.75,4.94 4.98,5.7 1.98,5.7 1.11,6.57 1.11,18.08 1.63,18.61 8.38,18.61 v8.5,18.48 | v8.47,17 8.5,16.97 U1.D38
  Vert 0.102: v8.5,18.48 8.47,18.45 v8.47,17
SPI_MOSI2  (via drill 0.2)
  Top 0.102: U1.D7 13,6.22 v12.74,5.97
  Horz 0.102: v12.74,5.97 12.18,5.4 8.5,5.4 8,5.9 6.44,5.9 v6.2,5.66
  Bottom 0.102: J2.62 5,3.34 5.16,3.5 5.16,3.77 5,3.93 5,5.5 5.16,5.66 v6.2,5.66
SPI_SCK
  Top 0.102: J2.57 6.25,4.18 6.41,4.35 6.41,4.85 5.15,6.11 2.14,6.11 1.52,6.74 1.52,17.92 1.8,18.2 8.03,18.2 8.28,17.95 8.72,17.95 8.97,18.2 9.8,18.2 10,18 U1.~D42
SPI_SCK2  (via drill 0.2)
  Top 0.102: v12,8.3 U1.~D5
  Bottom 0.102: J2.60 5.5,4.7 6.03,5.23 7.87,5.23 8.06,5.42 8.06,5.69 7.97,5.78 7.97,6.22 8.31,6.56 8.31,7.8 8.81,8.3 v12,8.3
SWDCK  (via drill 0.2)
  Top 0.102: J2.21 15.25,3.08 v15.2,3.08 | U1.SWDCK 7.5,9.95 v7.76,10.21
  Horz 0.102: v15.01,10.29 14.92,10.21 12.99,10.21 12.78,9.99 11.86,9.99 11.65,10.21 v7.76,10.21
  Vert 0.102: v15.01,10.29 15.2,10.1 15.2,6.01 15.42,5.79 15.42,5.51 15.2,5.29 v15.2,3.08
SWDIO
  Top 0.102: U1.SWDIO 11.5,5.8 11.72,5.58 13.46,5.58 13.76,5.29 13.76,3.95 14.75,2.95 J2.23
TX1
  Top 0.102: J2.17 16.25,1.98 16.09,2.14 16.09,2.41 16.25,2.57 16.25,4.48 15.41,5.32 14.96,5.32 14.5,5.78 U1.~D24
TXO-0  (via drill 0.2)
  Top 0.102: U1.TXO-0 v11,15.1
  Horz 0.102: v11,15.1 11.84,15.1 11.86,15.07 13.21,15.07 13.36,15.23 13.64,15.23 13.69,15.17 18.67,15.17 v18.8,15.3
  Bottom 0.102: v18.8,15.3 18.5,15 U6.9
USB_D+  (via drill 0.2)
  Top 0.102: J2.3 19.75,2.09 19.45,2.39 19.45,6.48 19.55,6.58 v19.55,7.11 v19.56,7.11
  Bottom 0.102: v19.56,7.11 19,7.67 U6.1
USB_D-  (via drill 0.2)
  Top 0.102: J2.5 19.25,6.68 v19.22,6.71
  Bottom 0.102: v19.22,6.71 18.5,7.43 U6.2

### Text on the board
Bottom: v10
Dimension: 45° Chamfered Edge
tDocu: 0.8mm PCB / 45 degree chamfered edge

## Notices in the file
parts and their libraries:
SparkFun-IC-Microcontroller: Licensing: Creative Commons ShareAlike 4.0 International - https://creativecommons.org/licenses/by-sa/4.0
SparkFun-Aesthetics: Released under the Creative Commons Attribution Share-Alike 4.0 License
SparkFun-Aesthetics: https://creativecommons.org/licenses/by-sa/4.0
